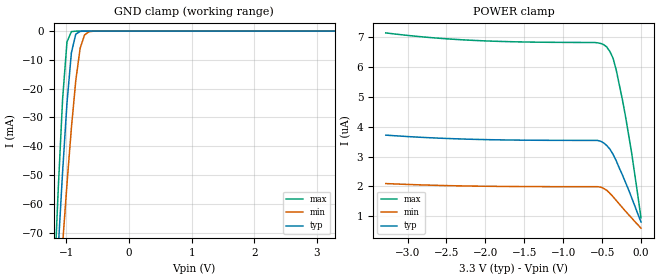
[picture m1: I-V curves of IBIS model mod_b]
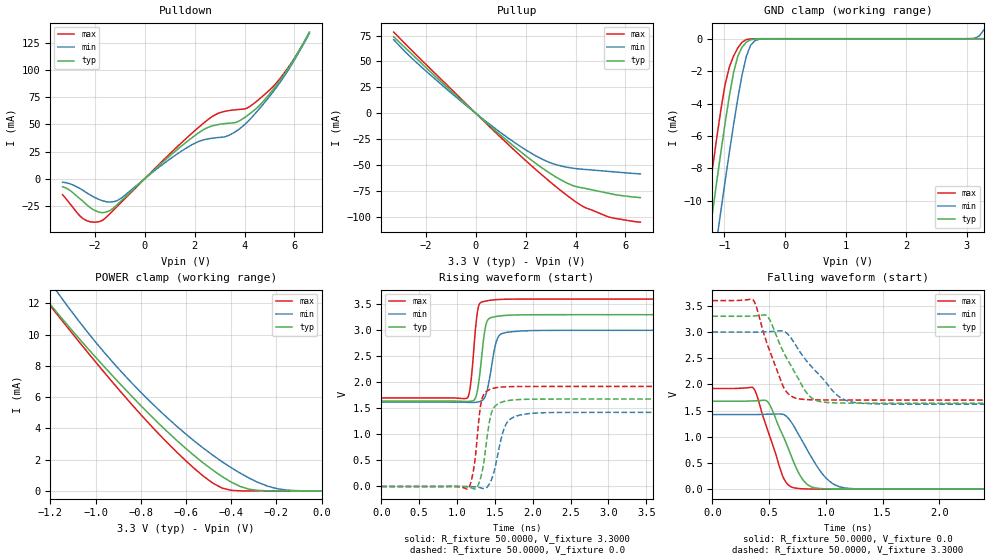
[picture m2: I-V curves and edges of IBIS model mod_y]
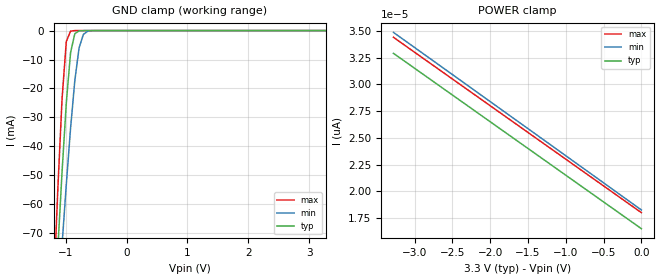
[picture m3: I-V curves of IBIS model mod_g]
| IBIS (I/O, Buffer, Information, Specification) Model, officially
| electronic behavioral standard for Buffer structures of digital pins.
[IBIS ver]  4.0
[File name] rhflvds32a_3v3_rev3.ibs
[File Rev]  3.0
[Date]   7 March 2018
[Source]   CAD & Design Services (Catania) - STMicroelectronics
[Notes]
   (Note1)  This IBIS model is the model of the product with package
   (Flat16 package elements);
   (Note2)  This IBIS model is extracted with nominal 3.3V power supply
   (min:3.0V, typ:3.3V, max:3.6V);
   (Note3)  This IBIS model has some Notes about the non-monotonicity
   of the I-V curves, but they are not indicative of problems
   inside the model;
[Disclaimer] Customers are solely responsible for all aspects of their
   own product designs or applications using this IBIS Model.
   STMicroelectronics assumes no liability for Custmer
   Designs and applications associated to this IBIS Model.
   In the use of this IBIS Model Customer shall not modify,
   disassemble, alter this Model in whole or in part.
   If Customers do not accept these terms, the IBIS Model
   may not be used. For any problems or modifications please
   contact STMicroelectronics (www.st.com).
[Copyright] (c) 2018 STMicroelectronics
|   Component RHFLVDS32A
[Component] RHFLVDS32A
[Manufacturer] STMicroelectronics
[Package]
| variable   typ   min   max
R_pkg   0.0   0.0   0.0
L_pkg   0.0H   0.0H   0.0H
C_pkg   0.0F   0.0F   0.0F
[Pin]   signal_name   model_name   R_pin   L_pin   C_pin
1   1B   mod_b   0.0   0.0   0.0
2   1A   mod_a   0.0   0.0   0.0
3   1Y   mod_y   0.0   0.0   0.0
4   G   mod_g   0.0   0.0   0.0
5   2Y   mod_y   0.0   0.0   0.0
6   2A   mod_a   0.0   0.0   0.0
7   2B   mod_b   0.0   0.0   0.0
8   GND   GND   0.0   0.0   0.0
9   3B   mod_b   0.0   0.0   0.0
10   3A   mod_a   0.0   0.0   0.0
11   3Y   mod_y   0.0   0.0   0.0
12   GN   mod_g   0.0   0.0   0.0
13   4Y   mod_y   0.0   0.0   0.0
14   4A   mod_a   0.0   0.0   0.0
15   4B   mod_b   0.0   0.0   0.0
16   VCC   POWER   0.0   0.0   0.0
[Diff pin]  inv_pin   vdiff   tdelay_typ  tdelay_min  tdelay_max
2   1   100mV   0.0s   0.0s   0.0s
6   7   100mV   0.0s   0.0s   0.0s
10   9   100mV   0.0s   0.0s   0.0s
14   15   100mV   0.0s   0.0s   0.0s
[Package Model]  292130_RHFLVDS32_IBIS
[Define Package Model]  292130_RHFLVDS32_IBIS
[Manufacturer]  STMicroelectronics
[OEM]  STMicroelectronics
[Description]  ceramic flat-16
[Number Of Pins] 16
[Pin Numbers]
|Pin Num   Terminal Name
1   | NET1:bwpad1_source
2   | NET2:bwpad2_source
3   | NET3:bwpad6_source
4   | NET4:bwpad7_source
5   | NET5:bwpad8_source
6   | NET6:bwpad12_source
7   | NET7:bwpad13_source
8   | NET8:net8_source
9   | NET9:bwpad19_source
10   | NET10:bwpad20_source
11   | NET11:bwpad24_source
12   | NET12:bwpad25_source
13   | NET13:bwpad26_source
14   | NET14:bwpad30_source
15   | NET15:bwpad31_source
16   | NET16:net16_source
[Model Data]
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[End Model Data]
[End Package Model]
| Models and submodels in the file (4): mod_b (Input), mod_a (Input), mod_y (3-state), mod_g (Input)
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|   Model mod_b
[Model]   mod_b
Model_type Input
Vinl   =   0.6500V
Vinh   =   1.2000V
C_comp   1.160pF   1.148pF   1.230pF
[Temperature Range]  25.0000   0.1250k   -55.0000
[Voltage Range]   3.3000V   3.0000V   3.6000V
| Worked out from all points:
|   GND clamp passes 1 mA (typ) near -0.85 V on its own axis
[GND_clamp]
|Voltage   I(typ)   I(min)   I(max)
-3.3V     -1.037A    -847.3mA   -1.291A
-1.2V     -103.9mA   -118.4mA   -90.61mA
-1.13V    -75.7mA    -95.97mA   -55.15mA
-1.06V    -48.92mA   -74.09mA   -23.64mA
-990mV    -24.98mA   -53.14mA   -3.768mA
-920mV    -7.585mA   -33.75mA   -179.6uA
-850mV    -1.057mA   -17.22mA   -5.053uA
-780mV    -97.1uA    -5.969mA   -122.7nA
-710mV    -6.82uA    -1.339mA   -2.974nA
-640mV    -449.9nA   -233.7uA   -80.51pA
-500mV    -1.943nA   -4.459uA   -7.043pA
3.28V     3.538uA    1.987uA    6.819uA
[POWER_clamp]
|Voltage   I(typ)   I(min)   I(max)
-3.28V    3.717uA    2.092uA    7.145uA
-2.24V    3.582uA    2.011uA    6.906uA
-560mV    3.539uA    1.988uA    6.813uA
-480mV    3.455uA    1.928uA    6.753uA
-440mV    3.369uA    1.867uA    6.673uA
-400mV    3.249uA    1.766uA    6.522uA
-360mV    3.079uA    1.654uA    6.302uA
-320mV    2.869uA    1.533uA    5.922uA
-240mV    2.389uA    1.289uA    4.922uA
-200mV    2.138uA    1.169uA    4.362uA
-120mV    1.618uA    937nA      3.121uA
0V        803nA      596.8nA    940.7nA
|   Model mod_y (*updated)
[Model]   mod_y
Model_type 3-state
Polarity   Non-Inverting
Enable   Active-High
Vmeas  =   1.650V
Cref   =   10pF
C_comp   0.703pF   0.691pF   0.736pF
[Temperature Range]  25.0000   0.1250k   -55.0000
[Voltage Range]   3.3000V   3.0000V   3.6000V
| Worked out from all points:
|   slope of the pulldown table from 0 to 0.495 V, typ, clamps not added: 46.8 ohm
|   slope of the pullup table from 0 to 0.495 V, typ, clamps not added: 46.7 ohm
|   GND clamp passes 1 mA (typ) near -0.77 V on its own axis
|   POWER clamp passes 1 mA (typ) near -0.45 V on its own axis
|   rising waveform, R_fixture 50.0000, V_fixture 3.3000: 20-80 % time 80.1ps typ, 102ps min, 69ps max; typ from 1.64 V to 3.3 V
|   rising waveform, R_fixture 50.0000, V_fixture 0.0: 20-80 % time 103ps typ, 140ps min, 84.5ps max; typ from 0 V to 1.68 V
|   falling waveform, R_fixture 50.0000, V_fixture 0.0: 20-80 % time 196ps typ, 238ps min, 172ps max; typ from 1.68 V to 0 V
|   falling waveform, R_fixture 50.0000, V_fixture 3.3000: 20-80 % time 235ps typ, 311ps min, 181ps max; typ from 3.3 V to 1.64 V
[Pulldown]
|Voltage   I(typ)   I(min)   I(max)
-3.3V     -7.537mA   -3.359mA   -14.98mA
-2.5V     -20.61mA   -10.57mA   -36.72mA
-1.7V     -31.46mA   -20.45mA   -38.52mA
-1V       -21.67mA   -18.82mA   -23.24mA
1V        20.92mA    17.92mA    22.83mA
2.2V      42.92mA    34.59mA    48.17mA
2.9V      49.73mA    37.79mA    59.83mA
3.6V      51.6mA     42.79mA    63.46mA
4.1V      57.96mA    51.95mA    65.07mA
5.1V      80.95mA    78.76mA    83.94mA
5.8V      103.5mA    101.9mA    104.2mA
6.6V      135.3mA    134.1mA    134.4mA
[Pullup]
|Voltage   I(typ)   I(min)   I(max)
-3.3V     73.83mA    71.03mA    78.3mA
-2.3V     50.9mA     47.2mA     54.13mA
-400mV    8.688mA    7.808mA    9.425mA
1.2V      -25.2mA    -22.13mA   -27.74mA
1.8V      -37.03mA   -32.07mA   -41.11mA
2.4V      -48.11mA   -40.83mA   -54.05mA
3V        -58.12mA   -47.67mA   -66.41mA
3.6V      -66.43mA   -51.65mA   -77.97mA
3.9V      -69.68mA   -52.84mA   -83.34mA
4.4V      -72.34mA   -54.03mA   -90.91mA
5.4V      -77.35mA   -56.03mA   -100.2mA
6.6V      -81.12mA   -58.23mA   -104.8mA
[GND_clamp]
|Voltage   I(typ)   I(min)   I(max)
-3.3V     -419.9mA   -358.7mA   -520.8mA
-1.34V    -14.67mA   -18.75mA   -12mA
-1.27V    -12.71mA   -16.47mA   -10.02mA
-1.2V     -10.78mA   -14.43mA   -8.069mA
-1.13V    -8.871mA   -12.5mA    -6.177mA
-1.06V    -7.008mA   -10.63mA   -4.39mA
-990mV    -5.213mA   -8.799mA   -2.835mA
-780mV    -1.074mA   -3.687mA   -566.7uA
-640mV    -214.8uA   -1.096mA   -51.51uA
-430mV    -2.51uA    -36.84uA   -49.01nA
3.07V     -1.212nA   5.416uA    -3.679pA
3.28V     -510.6pA   536.9uA    21.81pA
[POWER_clamp]
|Voltage   I(typ)   I(min)   I(max)
-3.28V    62.63mA    61.59mA    63.33mA
-1.24V    12.66mA    14.17mA    12.58mA
-1.16V    11.23mA    12.54mA    11.11mA
-960mV    7.923mA    8.839mA    7.561mA
-800mV    5.466mA    6.317mA    4.89mA
-600mV    2.707mA    3.631mA    1.92mA
-480mV    1.315mA    2.271mA    488.7uA
-440mV    915uA      1.866mA    180.9uA
-360mV    284.9uA    1.135mA    5.873uA
-240mV    7.695uA    311.4uA    14.93nA
-160mV    418.1nA    63.32uA    367.4pA
0V        144.8pA    43.49nA    68.82pA
[Ramp]
| variable   typ   min   max
dV/dt_r   1.0067/0.1407n   0.8543/0.1725n   1.1536/0.1285n
dV/dt_f   0.9964/0.2535n   0.8272/0.3241n   0.8760/0.4320n
R_load = 50.0000
[Rising Waveform]   |  updated
R_fixture= 50.0000
V_fixture= 3.3000
V_fixture_min= 3.0000
V_fixture_max= 3.6000
|time   V(typ)   V(min)   V(max)
0s        1.64V      1.621V     1.701V
1.138ns   1.632V     1.617V     1.704V
1.186ns   1.638V     1.615V     2.047V
1.258ns   1.764V     1.619V     3.23V
1.294ns   2.083V     1.629V     3.503V
1.366ns   2.991V     1.71V      3.558V
1.414ns   3.216V     1.955V     3.571V
1.522ns   3.267V     2.797V     3.589V
1.642ns   3.286V     2.956V     3.596V
6ns       3.3V       3V         3.6V
[Rising Waveform]   |  updated
R_fixture= 50.0000
V_fixture= 0.0
V_fixture_min= 0.0
V_fixture_max= 0.0
|time   V(typ)   V(min)   V(max)
0s        76.47nV    41.22uV    11.02nV
1.144ns   -12.22mV   253.5uV    -46.53mV
1.228ns   -47.58mV   -6.799mV   413.1mV
1.3ns     108.2mV    -20.59mV   1.442V
1.324ns   236.1mV    -30.34mV   1.654V
1.432ns   1.277V     60.94mV    1.863V
1.492ns   1.524V     302.8mV    1.89V
1.648ns   1.643V     1.199V     1.915V
1.876ns   1.673V     1.385V     1.921V
6ns       1.679V     1.424V     1.922V
[Falling Waveform]   |  updated
R_fixture= 50.0000
V_fixture= 0.0
V_fixture_min= 0.0
V_fixture_max= 0.0
|time   V(typ)   V(min)   V(max)
0s        1.679V     1.424V     1.922V
356ps     1.685V     1.424V     1.943V
386ps     1.688V     1.424V     1.829V
494ps     1.65V      1.431V     1.085V
626ps     1.005V     1.426V     220.5mV
734ps     429.7mV    1.144V     19.77mV
830ps     102.6mV    774.3mV    4.438mV
980ps     8.111mV    265.4mV    646.5uV
1.178ns   1.013mV    20.2mV     80.11uV
6ns       535.9nV    41.42uV    511.8nV
[Falling Waveform]   |  updated
R_fixture= 50.0000
V_fixture= 3.3000
V_fixture_min= 3.0000
V_fixture_max= 3.6000
|time   V(typ)   V(min)   V(max)
0s        3.3V       3V         3.6V
356ps     3.305V     2.999V     3.622V
488ps     3.292V     3.006V     2.742V
620ps     2.647V     3.02V      1.981V
680ps     2.406V     2.923V     1.799V
776ps     2.037V     2.608V     1.72V
920ps     1.69V      2.232V     1.704V
1.124ns   1.644V     1.755V     1.701V
1.304ns   1.641V     1.641V     1.701V
6ns       1.64V      1.621V     1.701V
|   Model mod_g
[Model]   mod_g
Model_type Input
Vinl   =   0.6500V
Vinh   =   1.2000V
C_comp   0.202pF   0.184pF   0.218pF
[Temperature Range]  25.0000   0.1250k   -55.0000
[Voltage Range]   3.3000V   3.0000V   3.6000V
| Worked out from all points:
|   GND clamp passes 1 mA (typ) near -0.85 V on its own axis
[GND_clamp]
|Voltage   I(typ)   I(min)   I(max)
-3.3V     -1.037A    -847.3mA   -1.291A
-1.2V     -103.9mA   -118.4mA   -90.61mA
-1.13V    -75.7mA    -95.97mA   -55.15mA
-1.06V    -48.91mA   -74.09mA   -23.64mA
-990mV    -24.98mA   -53.14mA   -3.767mA
-920mV    -7.584mA   -33.75mA   -179uA
-850mV    -1.056mA   -17.22mA   -4.994uA
-780mV    -96.57uA   -5.968mA   -121.2nA
-710mV    -6.743uA   -1.337mA   -2.93nA
-640mV    -444.3nA   -233uA     -73.86pA
-500mV    -1.914nA   -4.408uA   -2.541pA
3.28V     16.4pA     19.67pA    16.4pA
[POWER_clamp]
|Voltage   I(typ)   I(min)   I(max)
-3.28V    32.9pA     34.86pA    34.4pA
-2.44V    28.7pA     30.61pA    30.2pA
-1.4V     23.5pA     25.35pA    25pA
0V        16.5pA     18.25pA    18pA
